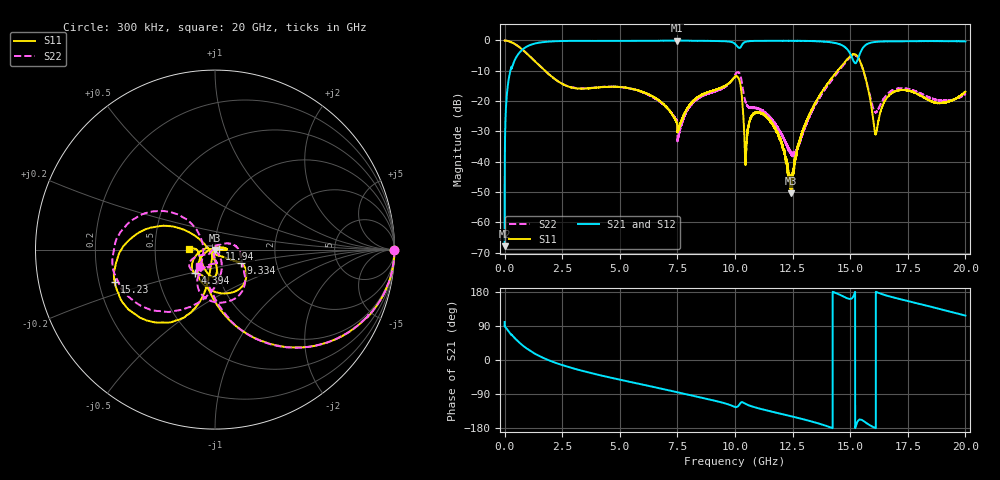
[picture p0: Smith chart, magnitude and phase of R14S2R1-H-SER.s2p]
!{R14S2R1}
!Johanson Technology Inc.
!www.johansontechnology.com
!Test Board Conditions:
!Substrate Type  RO4350B
!Substrate Thickness  20 mil
!Substrate Dk  3.66
!TL Type: GCPW
!TL Trace Width  36 mil
!TL Gap  12 mil
!Electrode orientation  Horizontal
!DUT TOPOLOGY	SERIES
!Mounting Pad LxW  26x36 mil
! Created Wed Nov 25 17:33:21 2020
! 2 Port Network Data from SP1.SP block
! freq  magS11  angS11  magS21  angS21  magS12  angS12  magS22  angS22
# khz S ma R 50
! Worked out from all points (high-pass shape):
!   20001 points, 300 kHz to 20 GHz, reference 50 ohm
!   highest |S21| = -0.05 dB at 7.47 GHz (marker M1); lowest = -67.9 dB at 300 kHz (marker M2)
!   |S21| within 3 dB of the highest: 769.3 MHz to 14.89 GHz (14.12 GHz wide, 180 % of centre); 15.5 GHz to end of sweep
!   lowest |S11| = -50.5 dB at 12.43 GHz (marker M3), VSWR 1.01, Z = 50.2 - j0.259 ohm
!   |S11| at or under -10 dB: 1.754 GHz to 14.45 GHz (12.7 GHz wide, 157 % of centre); 15.58 GHz to end of sweep
!   |S22| runs from -38.5 to 0.0 dB; largest |S21 - S12| = 0.015
!   S11 on the Smith chart (normalised r, x): 300 kHz: open; 4.394 GHz: 0.78, -0.21; 9.334 GHz: 1.32, -0.20; 11.94 GHz: 1.05, +0.00; 15.23 GHz: 0.27, -0.15; 20 GHz: 0.75, +0.01
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300  0.997 -0.1  0.0004038 100.3  0.0003563 100.2  0.9963 -0.2
131300  0.985 -10.9  0.1706 78.9  0.1712 78.9  0.9837 -10.9
484300  0.8546 -34.4  0.5109 55.1  0.5123 55.2  0.8548 -34.4
1517300  0.3845 -79.9  0.9196 10.4  0.9198 10.3  0.3853 -79.0
3334300  0.1602 -118.4  0.9833 -28.1  0.9834 -28.0  0.1621 -117.3
4394300  0.1709 -129.7  0.9808 -43.7  0.9807 -43.7  0.1726 -137.4
6667300  0.1047 -164.5  0.9895 -73.9  0.989 -73.8  0.1018 -159.6
7470300  0.04421 166.7  0.9942 -84.7  0.9925 -84.7  0.04805 -144.0
9334300  0.1622 -27.0  0.9757 -110.7  0.9766 -110.7  0.1542 -18.9
1.00003e7  0.253 -52.1  0.8778 -124.1  0.8766 -124.1  0.2707 -54.2
1.02283e7  0.1939 -113.5  0.7614 -114.2  0.7622 -114.2  0.2708 -103.1
1.04753e7  0.01224 59.5  0.9549 -116.3  0.9534 -116.3  0.09167 -112.0
1.09743e7  0.06532 1.3  0.9839 -126.7  0.9829 -126.7  0.07582 -82.5
1.19443e7  0.02395 3.4  0.9881 -141.4  0.9877 -141.3  0.03162 -99.4
1.24303e7  0.002997 -59.3  0.9844 -148.4  0.9872 -148.3  0.01349 -96.7
1.33343e7  0.07199 -106.5  0.9776 -162.5  0.9789 -162.4  0.06645 -59.9
1.48133e7  0.4609 -119.8  0.7544 164.5  0.7531 164.0  0.4419 -128.7
1.52293e7  0.588 -162.0  0.4199 -177.3  0.4192 -178.0  0.5676 -177.4
1.55433e7  0.3456 158.2  0.7464 -159.5  0.7426 -159.8  0.3395 141.4
1.60943e7  0.02899 -153.6  0.945 -179.5  0.9455 -179.5  0.06531 179.0
1.66673e7  0.1209 -84.8  0.9673 168.5  0.9637 168.5  0.1366 -131.5
2e7  0.1428 177.3  0.9627 117.1  0.9614 117.2  0.1305 -134.4
